| TEXAS INSTRUMENTS INCORPORATED
| Standard Linear and Logic Group
| IBIS Model of SN74CBT3257C
| 4 Bit 1-Of-2 FET Multiplexer/Demultiplexer with -2V Undershoot-Protection
| This file contains package information for the following:
|  SSOP 16-pin (DB) package as [Component] CBT3257C_DB
|  SOIC 16-pin (D) package as [Component] CBT3257C_D
|  TVSOP 16-pin (DGV) package as [Component] CBT3257C_DGV
|  TSSOP 16-pin (PW) package as [Component] CBT3257C_PW
|  SSOP 16-pin (DBQR) package as [Component] CBT3257C_DBQR
|  QFN 16-pin (RGY) package as [Component] CBT3257C_RGY
| This device can be powered at the following Vccs:
|  5 volt Vcc
|  4 volt Vcc
| This file provides unique models under the [Model Selector] for each Vcc.
| For operation at a specific Vcc, select the appropriate model after each
| [Model Selector] keyword.
[IBIS Ver]   3.2
[Comment char]  |_char
[File Name]   sn74cbt3257c.ibs
[File Rev]   1.1 | b_die
[Date]   June 23, 2003
[Source]   Data created from TI-SPICE simulations at TI-SLL.
[Notes]   The following is an IBIS list for the CBT3257C.
   Please contact sllibis@ti.com with questions and
   comments concerning SLL IBIS models.
   -Non-monotonic data due to FET characteristics.
   -Power clamp data deleted as there is no power-clamp diode.
[Disclaimer] Property of Texas Instruments Incorporated.  Unauthorized
   reproduction and/or distribution is strictly prohibited.
   This product is protected under copyright law.
   Created  2003, (C) Copyright  2003, Texas Instruments
   Incorporated, All Rights Reserved
   UNLESS THERE IS A SIGNED, WRITTEN AGREEMENT TO THE
   CONTRARY, TEXAS INSTRUMENTS (TI) IS PROVIDING THE IBIS
   MODELS  AND WITHOUT ANY WARRANTY, EXPRESSED OR
   IMPLIED.  TI assumes no liability for:
   1) the accuracy of the IBIS models provided to your
   company;
   2) the proper functioning of these IBIS Models in your
   design or for any resulting applications; or
   3) infringement of patents, copyrights or intellectual
   property rights resulting from your use of these IBIS
   models.
   TI provides IBIS Models as a service to our customers.
   You and your company shall not distribute, sell or give
   these models to anyone else without prior written
   permission from TI.
   TI reserves the right to make changes to our products or
   to discontinue any semiconductor product or service
   without notice, and advises our customers to obtain the
   latest version of relevant information to verify, before
   placing orders, that the information being relied on is
   current.
   Please be aware that your receipt and use of the IBIS
   information provided shall serve as acceptance of these
   terms and conditions.  If you do not accept these terms,
   you should return or destroy the IBIS models and any
   other accompanying information immediately.
| Component CBT3257C_D 16-pin SOIC
[Component]   CBT3257C_D
[Manufacturer]   Texas Instruments, Inc.
[Package]
|   typ   min   max
R_pkg   3.900e-02   2.800e-02   4.900e-02
L_pkg   3.453e-09   2.350e-09   4.375e-09
C_pkg   5.210e-13   2.540e-13   7.080e-13
[Pin]   signal_name   model_name   R_pin   L_pin   C_pin
1   S   CBT3257C_IN   4.200e-02   4.336e-09   7.030e-13
2   1B1   CBT3257C_IO   4.900e-02   3.778e-09   6.340e-13
3   1B2   CBT3257C_IO   2.800e-02   3.449e-09   5.180e-13
4   1A   CBT3257C_IO   2.900e-02   2.393e-09   2.540e-13
5   2B1   CBT3257C_IO   2.800e-02   2.350e-09   2.640e-13
6   2B2   CBT3257C_IO   4.800e-02   3.312e-09   4.830e-13
7   2A   CBT3257C_IO   4.300e-02   3.629e-09   6.040e-13
8   GND   GND   4.400e-02   4.375e-09   7.080e-13
9   3A   CBT3257C_IO   4.200e-02   4.336e-09   7.030e-13
10   3B2   CBT3257C_IO   4.900e-02   3.778e-09   6.340e-13
11   3B1   CBT3257C_IO   2.800e-02   3.449e-09   5.180e-13
12   4A   CBT3257C_IO   2.900e-02   2.393e-09   2.550e-13
13   4B2   CBT3257C_IO   2.800e-02   2.350e-09   2.640e-13
14   4B1   CBT3257C_IO   4.800e-02   3.312e-09   4.830e-13
15   NOE   CBT3257C_IN   4.300e-02   3.629e-09   6.040e-13
16   VCC   POWER   4.400e-02   4.375e-09   7.080e-13
| Component CBT3257C_DB 16-pin SSOP
[Component]   CBT3257C_DB
[Manufacturer]   Texas Instruments, Inc.
[Package]
|   typ   min   max
R_pkg   4.800e-02   4.600e-02   5.000e-02
L_pkg   3.536e-09   3.213e-09   3.798e-09
C_pkg   3.760e-13   3.140e-13   4.400e-13
[Pin]   signal_name   model_name   R_pin   L_pin   C_pin
1   S   CBT3257C_IN   4.800e-02   3.797e-09   3.770e-13
2   1B1   CBT3257C_IO   4.600e-02   3.723e-09   4.400e-13
3   1B2   CBT3257C_IO   4.800e-02   3.409e-09   3.720e-13
4   1A   CBT3257C_IO   4.900e-02   3.213e-09   3.140e-13
5   2B1   CBT3257C_IO   4.900e-02   3.213e-09   3.140e-13
6   2B2   CBT3257C_IO   4.800e-02   3.409e-09   3.720e-13
7   2A   CBT3257C_IO   4.600e-02   3.723e-09   4.400e-13
8   GND   GND   4.800e-02   3.798e-09   3.770e-13
9   3A   CBT3257C_IO   4.800e-02   3.797e-09   3.770e-13
10   3B2   CBT3257C_IO   4.600e-02   3.725e-09   4.400e-13
11   3B1   CBT3257C_IO   4.800e-02   3.409e-09   3.720e-13
12   4A   CBT3257C_IO   4.900e-02   3.214e-09   3.140e-13
13   4B2   CBT3257C_IO   5.000e-02   3.216e-09   3.140e-13
14   4B1   CBT3257C_IO   4.800e-02   3.409e-09   3.720e-13
15   NOE   CBT3257C_IN   4.700e-02   3.729e-09   4.400e-13
16   VCC   POWER   4.800e-02   3.797e-09   3.770e-13
| Component CBT3257C_DGV 16-pin TVSOP
[Component]   CBT3257C_DGV
[Manufacturer]   Texas Instruments, Inc.
[Package]
|   typ   min   max
R_pkg   3.900e-02   3.300e-02   4.500e-02
L_pkg   2.543e-09   2.320e-09   2.938e-09
C_pkg   3.860e-13   3.340e-13   4.490e-13
[Pin]   signal_name   model_name   R_pin   L_pin   C_pin
1   S   CBT3257C_IN   3.500e-02   2.907e-09   4.170e-13
2   1B1   CBT3257C_IO   4.200e-02   2.558e-09   4.460e-13
3   1B2   CBT3257C_IO   3.800e-02   2.341e-09   3.450e-13
4   1A   CBT3257C_IO   3.800e-02   2.320e-09   3.340e-13
5   2B1   CBT3257C_IO   3.900e-02   2.322e-09   3.340e-13
6   2B2   CBT3257C_IO   3.800e-02   2.353e-09   3.420e-13
7   2A   CBT3257C_IO   4.000e-02   2.536e-09   4.410e-13
8   GND   GND   3.300e-02   2.897e-09   4.180e-13
9   3A   CBT3257C_IO   3.500e-02   2.927e-09   4.190e-13
10   3B2   CBT3257C_IO   4.500e-02   2.632e-09   4.490e-13
11   3B1   CBT3257C_IO   3.900e-02   2.368e-09   3.470e-13
12   4A   CBT3257C_IO   3.900e-02   2.330e-09   3.350e-13
13   4B2   CBT3257C_IO   3.900e-02   2.320e-09   3.350e-13
14   4B1   CBT3257C_IO   3.900e-02   2.361e-09   3.450e-13
15   NOE   CBT3257C_IN   4.100e-02   2.573e-09   4.460e-13
16   VCC   POWER   3.500e-02   2.938e-09   4.200e-13
| Component CBT3257C_PW 16-pin TSSOP
[Component]   CBT3257C_PW
[Manufacturer]   Texas Instruments, Inc.
[Package]
|   typ   min   max
R_pkg   4.500e-02   3.800e-02   5.100e-02
L_pkg   2.593e-09   2.447e-09   3.080e-09
C_pkg   2.810e-13   2.430e-13   3.770e-13
[Pin]   signal_name   model_name   R_pin   L_pin   C_pin
1   S   CBT3257C_IN   4.000e-02   3.080e-09   3.770e-13
2   1B1   CBT3257C_IO   3.800e-02   2.458e-09   2.810e-13
3   1B2   CBT3257C_IO   5.100e-02   2.512e-09   2.550e-13
4   1A   CBT3257C_IO   5.100e-02   2.447e-09   2.430e-13
5   2B1   CBT3257C_IO   5.100e-02   2.447e-09   2.430e-13
6   2B2   CBT3257C_IO   5.100e-02   2.512e-09   2.550e-13
7   2A   CBT3257C_IO   3.800e-02   2.458e-09   2.810e-13
8   GND   GND   4.000e-02   3.080e-09   3.770e-13
9   3A   CBT3257C_IO   3.900e-02   2.832e-09   3.160e-13
10   3B2   CBT3257C_IO   3.800e-02   2.460e-09   2.790e-13
11   3B1   CBT3257C_IO   5.100e-02   2.512e-09   2.550e-13
12   4A   CBT3257C_IO   5.100e-02   2.447e-09   2.430e-13
13   4B2   CBT3257C_IO   5.100e-02   2.447e-09   2.430e-13
14   4B1   CBT3257C_IO   5.100e-02   2.512e-09   2.550e-13
15   NOE   CBT3257C_IN   3.800e-02   2.459e-09   2.790e-13
16   VCC   POWER   3.900e-02   2.832e-09   3.160e-13
| Component CBT3257C_DBQR 16-pin SSOP
[Component]   CBT3257C_DBQR
[Manufacturer]   Texas Instruments, Inc.
[Package]
|   typ   min   max
R_pkg   3.800e-02   2.700e-02   5.900e-02
L_pkg   2.353e-09   1.491e-09   4.500e-09
C_pkg   2.100e-13   6.400e-14   5.920e-13
[Pin]   signal_name   model_name   R_pin   L_pin   C_pin
1   S   CBT3257C_IN   5.800e-02   4.450e-09   5.920e-13
2   1B1   CBT3257C_IO   4.000e-02   1.930e-09   1.110e-13
3   1B2   CBT3257C_IO   2.800e-02   1.538e-09   7.600e-14
4   1A   CBT3257C_IO   2.700e-02   1.491e-09   6.400e-14
5   2B1   CBT3257C_IO   2.700e-02   1.491e-09   6.400e-14
6   2B2   CBT3257C_IO   2.700e-02   1.506e-09   7.500e-14
7   2A   CBT3257C_IO   3.300e-02   1.922e-09   1.090e-13
8   GND   GND   5.900e-02   4.500e-09   5.880e-13
9   3A   CBT3257C_IO   5.800e-02   3.695e-09   4.140e-13
10   3B2   CBT3257C_IO   3.400e-02   2.685e-09   2.820e-13
11   3B1   CBT3257C_IO   2.900e-02   1.552e-09   7.700e-14
12   4A   CBT3257C_IO   2.800e-02   1.506e-09   6.500e-14
13   4B2   CBT3257C_IO   2.700e-02   1.492e-09   6.400e-14
14   4B1   CBT3257C_IO   2.800e-02   1.534e-09   7.600e-14
15   NOE   CBT3257C_IN   4.000e-02   2.703e-09   2.840e-13
16   VCC   POWER   5.600e-02   3.645e-09   4.180e-13
| Component CBT3257C_RGY 16-pin QFN
[Component]   CBT3257C_RGY
[Manufacturer]   Texas Instruments, Inc.
[Package]
|   typ   min   max
R_pkg   3.000e-02   2.700e-02   3.800e-02
L_pkg   8.000e-10   7.220e-10   9.400e-10
C_pkg   1.410e-13   1.290e-13   1.550e-13
[Pin]   signal_name   model_name   R_pin   L_pin   C_pin
1   S   CBT3257C_IN   2.700e-02   8.180e-10   1.320e-13
2   1B1   CBT3257C_IO   2.700e-02   8.030e-10   1.300e-13
3   1B2   CBT3257C_IO   3.700e-02   9.080e-10   1.500e-13
4   1A   CBT3257C_IO   2.900e-02   7.220e-10   1.390e-13
5   2B1   CBT3257C_IO   2.900e-02   7.220e-10   1.390e-13
6   2B2   CBT3257C_IO   2.900e-02   7.300e-10   1.400e-13
7   2A   CBT3257C_IO   2.900e-02   7.240e-10   1.390e-13
8   GND   GND   3.100e-02   8.000e-10   1.400e-13
9   3A   CBT3257C_IO   2.700e-02   8.110e-10   1.290e-13
10   3B2   CBT3257C_IO   2.800e-02   7.840e-10   1.310e-13
11   3B1   CBT3257C_IO   3.700e-02   9.150e-10   1.530e-13
12   4A   CBT3257C_IO   2.900e-02   8.470e-10   1.520e-13
13   4B2   CBT3257C_IO   2.900e-02   7.580e-10   1.430e-13
14   4B1   CBT3257C_IO   2.900e-02   7.720e-10   1.440e-13
15   NOE   CBT3257C_IN   2.900e-02   7.400e-10   1.420e-13
16   VCC   POWER   3.800e-02   9.400e-10   1.550e-13
[Series Switch Groups]
| Function Group States
On  1 /   | 1A->1B1 NOE LOW, S LOW
On  2 /   | 2A->2B1 NOE LOW, S LOW
On  3 /   | 3A->3B1 NOE LOW, S LOW
On  4 /   | 4A->4B1 NOE LOW, S LOW
On  5 /   | 1A->1B2 NOE LOW, S HIGH
On  6 /   | 2A->2B2 NOE LOW, S HIGH
On  7 /   | 3A->3B2 NOE LOW, S HIGH
On  8 /   | 4A->4B2 NOE LOW, S HIGH
On  1 2 3 4  /   | ENABLE 1B1 2B1 3B1 4B1
On  5 6 7 8 /   | ENABLE 1B2 2B2 3B2 4B2
Off 1 2 3 4 5 6 7 8  / | DISABLE ALL
[Series Pin Mapping]   pin_2   model_name   function_table_group
4   2   CBT3257C_IO_50_S   1
| 4   2   CBT3257C_IO_40_S   1
7   5   CBT3257C_IO_50_S   2
| 7   5   CBT3257C_IO_40_S   2
9   11   CBT3257C_IO_50_S   3
| 9   11   CBT3257C_IO_40_S   3
12   14   CBT3257C_IO_50_S   4
| 12   14   CBT3257C_IO_40_S   4
4   3   CBT3257C_IO_50_S   5
| 4   3   CBT3257C_IO_40_S   5
7   6   CBT3257C_IO_50_S   6
| 7   6   CBT3257C_IO_40_S   6
9   10   CBT3257C_IO_50_S   7
| 9   10   CBT3257C_IO_40_S   7
12   13   CBT3257C_IO_50_S   8
| 12   13   CBT3257C_IO_40_S   8
| Model CBT3257C_IN
[Model Selector]   CBT3257C_IN
CBT3257C_IN_50   5 volt Vcc
CBT3257C_IN_40   4 volt Vcc
| Model CBT3257C_IO
[Model Selector]   CBT3257C_IO
CBT3257C_IO_50   5 volt Vcc
CBT3257C_IO_40   4 volt Vcc
| Model CBT3257C_IO_S
[Model Selector]   CBT3257C_IO_S
CBT3257C_IO_50_S   5 volt Vcc
CBT3257C_IO_40_S   4 volt Vcc
[Model]   CBT3257C_IO_50_S
Model_type  Series_switch
| variable   typ   min   max
C_comp   0   0   0
[Temperature Range]   40   100   -40
| Ambient temperature   25   85   -40
[Voltage range]   5   4.5   5.5
[On]
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[Off]
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[Model]   CBT3257C_IO_40_S
Model_type  Series_switch
| variable   typ   min   max
C_comp   0   0   0
[Temperature Range]   40   100   -40
| Ambient temperature   25   85   -40
[Voltage range]   4   4   4
[On]
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[Off]
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| Models and submodels in the file (6): CBT3257C_IN_50 (Input), CBT3257C_IN_40 (Input), CBT3257C_IO_50_S (Series_switch), CBT3257C_IO_50 (Terminator), CBT3257C_IO_40_S (Series_switch), CBT3257C_IO_40 (Terminator)
